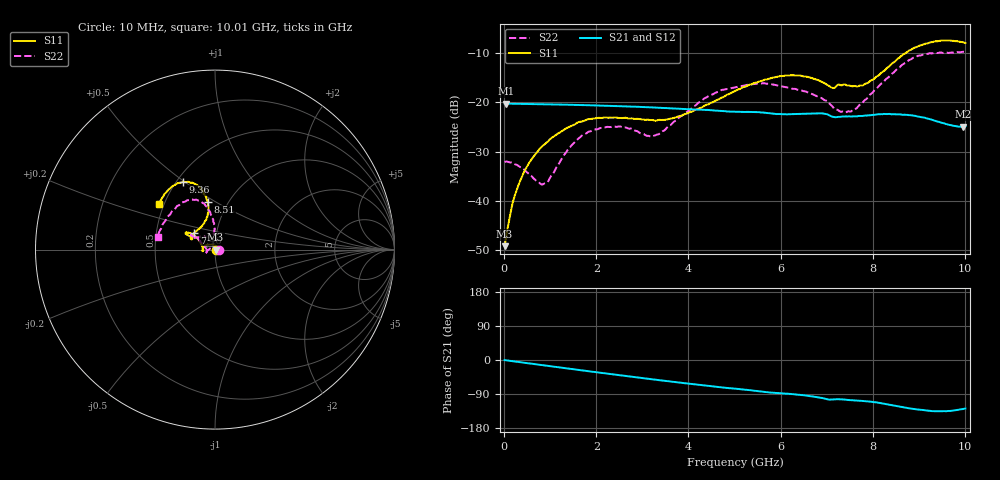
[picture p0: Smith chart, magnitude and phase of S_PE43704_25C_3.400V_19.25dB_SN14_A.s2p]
! Device ID: PE43704
! Dir: z:\PE43704\PE43704_Char_1_20130516\PE43704\AMB\3p400V\19p25dB
! Serial: 14
! Insertion: A
! Impedance: 50 ohm
! Temp: Amb
! VDD: 3.400V
! Attenuation Step: 19.25dB
! IDD: 1.140682e-01mA
#  Hz  S  RI  R  50
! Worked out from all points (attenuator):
!   401 points, 10 MHz to 10.01 GHz, reference 50 ohm
!   highest |S21| = -20.23 dB at 35 MHz (marker M1); lowest = -24.9 dB at 9.96 GHz (marker M2)
!   lowest |S11| = -49.1 dB at 10 MHz (marker M3), VSWR 1.01, Z = 50.3 + j0.0483 ohm
!   |S11| at or under -10 dB: start of sweep to 8.715 GHz
!   |S22| runs from -36.6 to -9.7 dB; largest |S21 - S12| = 0.001
!   S11 on the Smith chart (normalised r, x): 10 MHz: 1.01, +0.00; 7.46 GHz: 0.78, +0.15; 8.51 GHz: 0.81, +0.46; 9.36 GHz: 0.54, +0.49; 10.01 GHz: 0.47, +0.28
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1e7  0.00346 0.000479  0.0973 -0.000316  0.0974 -0.000267  0.025 0.000174
3.5e7  0.00364 0.0018  0.0973 -0.00108  0.0974 -0.0011  0.0251 0.00093
2.35e8  0.00163 0.0114  0.0967 -0.00677  0.0967 -0.00676  0.0225 0.00711
5.6e8  -0.00782 0.0238  0.0952 -0.0156  0.0952 -0.0156  0.0121 0.014
9.1e8  -0.025 0.0296  0.0926 -0.0247  0.0926 -0.0247  -0.00589 0.0141
1.385e9  -0.0505 0.0241  0.0876 -0.0364  0.0876 -0.0364  -0.0333 0.00208
1.685e9  -0.0621 0.0152  0.0835 -0.0433  0.0836 -0.0432  -0.0451 -0.00949
2.36e9  -0.07 -0.00375  0.0727 -0.0565  0.0727 -0.0565  -0.0515 -0.0242
3.36e9  -0.0666 -0.000576  0.053 -0.0707  0.0529 -0.0706  -0.0477 0.00269
4.41e9  -0.0844 0.0437  0.0314 -0.078  0.0314 -0.078  -0.0953 0.0623
5.01e9  -0.1085 0.0721  0.0199 -0.0781  0.0202 -0.0781  -0.1218 0.0734
5.96e9  -0.1563 0.0958  0.00333 -0.0763  0.00359 -0.0761  -0.1278 0.0736
6.685e9  -0.1563 0.0824  -0.00821 -0.0769  -0.0083 -0.0767  -0.1012 0.0674
7.11e9  -0.1254 0.0648  -0.0176 -0.0698  -0.0178 -0.0697  -0.0571 0.073
7.46e9  -0.1148 0.0942  -0.0191 -0.0695  -0.0188 -0.0696  -0.0235 0.0778
7.835e9  -0.0683 0.1383  -0.0236 -0.0699  -0.0233 -0.0696  -0.0037 0.1065
8.36e9  -0.0362 0.2305  -0.0359 -0.0676  -0.0355 -0.0675  -0.016 0.1835
8.51e9  -0.039 0.2662  -0.0397 -0.0647  -0.0392 -0.0648  -0.0286 0.2119
8.935e9  -0.0891 0.3514  -0.0471 -0.0558  -0.0467 -0.0554  -0.0946 0.2733
9.36e9  -0.1789 0.3776  -0.0462 -0.0457  -0.0465 -0.0458  -0.1863 0.2599
9.96e9  -0.3042 0.2722  -0.0359 -0.0438  -0.0363 -0.0439  -0.3133 0.0929
1.001e10  -0.3117 0.2525  -0.0354 -0.0451  -0.0361 -0.045  -0.3191 0.0714
